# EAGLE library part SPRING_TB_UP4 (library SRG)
Spring loaded Terminal block 4UCON 0.10 pitch straight (wire goes in top) 2 amps 20-26 AWG Adafruit: P/N 1081
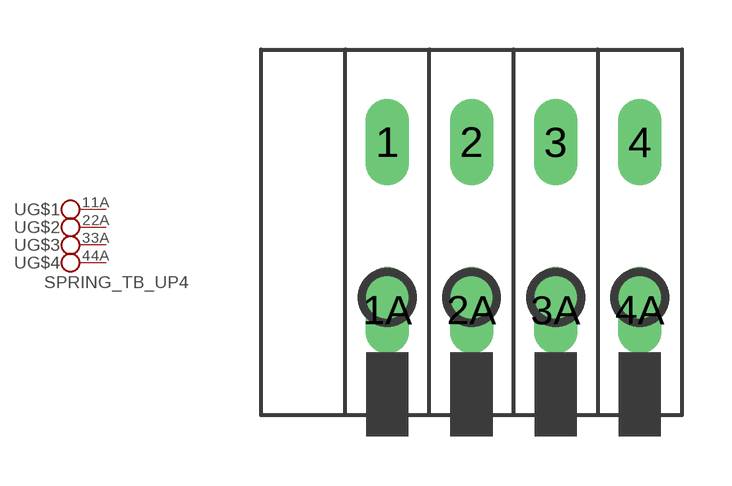
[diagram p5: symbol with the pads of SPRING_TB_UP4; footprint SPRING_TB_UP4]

Designator prefix -; gates G$1=KL2 G$2=KL2 G$3=KL2 G$4=KL2V

## SPRING_TB_UP4  [SPRING_TB_UP4]
1  G$1:1  pas
1A  G$1:2  pas
2  G$2:1  pas
2A  G$2:2  pas
3  G$3:1  pas
3A  G$3:2  pas
4  G$4:1  pas
4A  G$4:2  pas

## Footprint SPRING_TB_UP4 (pad centres in mm)
Spring Loaded Terminal Block 4UCON 0.10 pitch straight (wire goes in top) 2 amps 20-26 AWG Adafruit: P/N 1081 Terminal block comes with 3 terminals, but the are modular so you can add or remove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
drill 0.8 long: 1 -3.81,2.54; 1A -3.81,-2.54; 2 -1.27,2.54; 2A -1.27,-2.54; 3 1.27,2.54; 3A 1.27,-2.54; 4 3.81,2.54; 4A 3.81,-2.54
